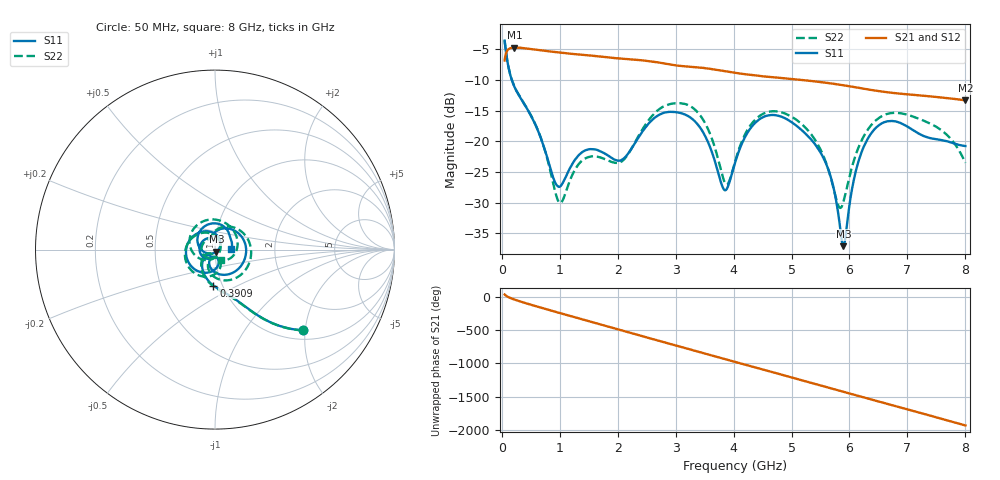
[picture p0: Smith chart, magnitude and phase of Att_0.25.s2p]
#  HZ  S  DB  R  50.00
! Rohde & Schwarz Vector Network Analyzer
! Rohde-Schwarz,ZNB40-4Port,1311601084101679,3.45
! Created: UTC 4/25/2025, 9:27:13 AM
! freq[Hz]  db:S11  ang:S11  db:S21  ang:S21  db:S12  ang:S12  db:S22  ang:S22
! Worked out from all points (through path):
!   1750 points, 50 MHz to 8 GHz, reference 50 ohm
!   highest |S21| = -4.69 dB at 218.2 MHz (marker M1); lowest = -13.3 dB at 8 GHz (marker M2)
!   group delay of S21, straight-line fit = 669 ps
!   lowest |S11| = -37.1 dB at 5.895 GHz (marker M3), VSWR 1.03, Z = 50.8 - j1.14 ohm
!   |S11| at or under -10 dB: 174.7 MHz to end of sweep
!   |S22| runs from -30.9 to -3.5 dB; largest |S21 - S12| = 0.00072
!   S11 on the Smith chart (normalised r, x): 50 MHz: 1.20, -1.94; 390.9 MHz: 0.91, -0.38; 8 GHz: 1.20, +0.01
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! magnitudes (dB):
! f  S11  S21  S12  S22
! 50 MHz  -3.6  -6.8  -6.8  -3.5
! 218.2 MHz  -11.1  -4.7  -4.7  -11.0
! 390.9 MHz  -14.0  -4.8  -4.8  -13.9
! 672.7 MHz  -19.4  -5.1  -5.1  -19.4
! 990.9 MHz  -27.4  -5.5  -5.5  -30.0
! 1.377 GHz  -21.9  -5.9  -5.9  -23.2
! 2.068 GHz  -23.0  -6.5  -6.5  -23.3
! 2.7 GHz  -15.8  -7.1  -7.1  -14.9
! 3.373 GHz  -17.1  -7.9  -7.9  -15.2
! 3.845 GHz  -28.0  -8.5  -8.5  -26.7
! 4.027 GHz  -23.4  -8.8  -8.8  -23.2
! 4.264 GHz  -18.2  -9.1  -9.1  -17.8
! 4.564 GHz  -15.8  -9.4  -9.4  -15.3
! 5.35 GHz  -19.8  -10.2  -10.2  -19.0
! 5.664 GHz  -25.4  -10.5  -10.5  -25.5
! 5.809 GHz  -32.0  -10.7  -10.7  -30.5
! 5.895 GHz  -37.1  -10.8  -10.8  -29.9
! 6.068 GHz  -26.6  -11.1  -11.1  -23.4
! 6.209 GHz  -21.8  -11.3  -11.3  -19.9
! 6.677 GHz  -16.7  -12.0  -12.0  -15.5
! 7.518 GHz  -19.7  -12.8  -12.8  -17.7
! 8 GHz  -20.8  -13.3  -13.3  -23.5
